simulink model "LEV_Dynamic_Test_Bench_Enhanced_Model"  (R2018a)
settings: Solver=VariableStepAuto  StartTime=0  StopTime=100  RelTol=1e-3
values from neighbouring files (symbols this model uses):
  Anglog_Input_Max = 10    [Panda_BEVintage_VPE_S_Data_Enhanced_Model.m]    (also in ParameterInitializationFileFinal.m = 3; Panda_BEVintage_VPE_S_Data_CodeGen_Model.m)
  Anglog_Input_Min = -10    [Panda_BEVintage_VPE_S_Data_Enhanced_Model.m]    (also in ParameterInitializationFileFinal.m = 0; Panda_BEVintage_VPE_S_Data_CodeGen_Model.m)
  Anglog_Output_Max = 10    [Panda_BEVintage_VPE_S_Data_Enhanced_Model.m]    (also in Panda_BEVintage_VPE_S_Data_CodeGen_Model.m)
  Anglog_Output_Min = -10    [Panda_BEVintage_VPE_S_Data_Enhanced_Model.m]    (also in Panda_BEVintage_VPE_S_Data_CodeGen_Model.m)
  Bits = 16    [Panda_BEVintage_VPE_S_Data_Enhanced_Model.m]    (also in ParameterInitializationFileFinal.m = 12; Panda_BEVintage_VPE_S_Data_CodeGen_Model.m)
  c_1 = 0    [Panda_BEVintage_VPE_S_Data_Enhanced_Model.m]    (also in Panda_BEVintage_VPE_S_Data_CodeGen_Model.m)
  FOH_Time = 0.001    [Panda_BEVintage_VPE_S_Data_Enhanced_Model.m]    (also in Panda_BEVintage_VPE_S_Data_CodeGen_Model.m)
  Full_BTrq_Range = Max_BTrq-Min_BTrq    (= 132)    [Panda_BEVintage_VPE_S_Data_Enhanced_Model.m]    (also in Panda_BEVintage_VPE_S_Data_CodeGen_Model.m)
  Full_Scale_Reading = Anglog_Input_Max-Anglog_Input_Min    (= 20)    [Panda_BEVintage_VPE_S_Data_Enhanced_Model.m]    (also in ParameterInitializationFileFinal.m = 3; Panda_BEVintage_VPE_S_Data_CodeGen_Model.m)
  Full_Speed_Range = Max_Speed-Min_Speed    (= 2513.27412287)    [Panda_BEVintage_VPE_S_Data_Enhanced_Model.m]    (also in Panda_BEVintage_VPE_S_Data_CodeGen_Model.m)
  g = 9.81    [Panda_BEVintage_VPE_S_Data_Enhanced_Model.m]    (also in Panda_BEVintage_VPE_S_Data_CodeGen_Model.m)
  m_e = 1.0359e+03    (= 1035.9)    [Panda_BEVintage_VPE_S_Data_Enhanced_Model.m]    (also in Panda_BEVintage_VPE_S_Data_CodeGen_Model.m)
  Max_BTrq = T_m_max    (= 66)    [Panda_BEVintage_VPE_S_Data_Enhanced_Model.m]    (also in Panda_BEVintage_VPE_S_Data_CodeGen_Model.m)
  Max_Speed = 400*pi    (= 1256.63706144)    [Panda_BEVintage_VPE_S_Data_Enhanced_Model.m]    (also in Panda_BEVintage_VPE_S_Data_CodeGen_Model.m)
  MaxInputBTrq = 5    [Panda_BEVintage_VPE_S_Data_Enhanced_Model.m]    (also in Panda_BEVintage_VPE_S_Data_CodeGen_Model.m)
  MaxOutputSpeedSensor = 5    [Panda_BEVintage_VPE_S_Data_Enhanced_Model.m]    (also in Panda_BEVintage_VPE_S_Data_CodeGen_Model.m)
  Min_BTrq = -T_m_max    (= -66)    [Panda_BEVintage_VPE_S_Data_Enhanced_Model.m]    (also in Panda_BEVintage_VPE_S_Data_CodeGen_Model.m)
  Min_Speed = -400*pi    (= -1256.63706144)    [Panda_BEVintage_VPE_S_Data_Enhanced_Model.m]    (also in Panda_BEVintage_VPE_S_Data_CodeGen_Model.m)
  MinInputBTrq = -5    [Panda_BEVintage_VPE_S_Data_Enhanced_Model.m]    (also in Panda_BEVintage_VPE_S_Data_CodeGen_Model.m)
  MinOutputSpeedSensor = -5    [Panda_BEVintage_VPE_S_Data_Enhanced_Model.m]    (also in Panda_BEVintage_VPE_S_Data_CodeGen_Model.m)
  r_e = 0.27    [Panda_BEVintage_VPE_S_Data_Enhanced_Model.m]    (also in Panda_BEVintage_VPE_S_Data_CodeGen_Model.m)
  Sampling_Time = 0.0001    [Panda_BEVintage_VPE_S_Data_Enhanced_Model.m]    (also in ParameterInitializationFileFinal.m = 0.01; Panda_BEVintage_VPE_S_Data_CodeGen_Model.m)
  T_m_max = 66    [Panda_BEVintage_VPE_S_Data_Enhanced_Model.m]    (also in Panda_BEVintage_VPE_S_Data_CodeGen_Model.m)
  T_r = 8.67    [Panda_BEVintage_VPE_S_Data_Enhanced_Model.m]    (also in Panda_BEVintage_VPE_S_Data_CodeGen_Model.m)
  ZOH_Time = 0.0001    [Panda_BEVintage_VPE_S_Data_Enhanced_Model.m]    (also in Panda_BEVintage_VPE_S_Data_CodeGen_Model.m)
undefined symbols (not defined in the file or in its folder): m, s, seconds
libraries: simulink x3, autolibmappedmotor x2, autolibshared x2, autolibsharedcoupling x1

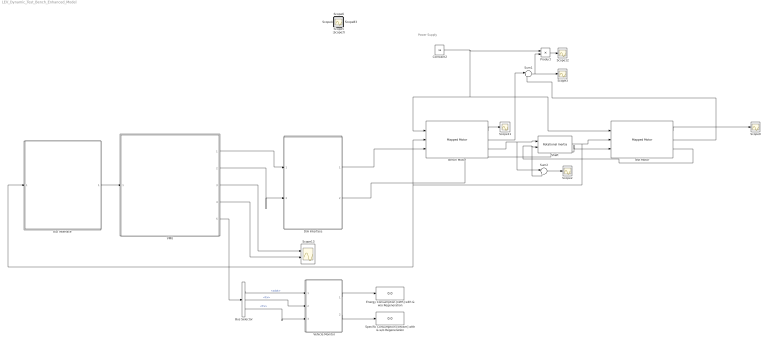
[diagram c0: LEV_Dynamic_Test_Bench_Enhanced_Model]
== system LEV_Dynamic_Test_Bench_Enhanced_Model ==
  note: Power Supply
  "A/D Interface " : Subsystem
  Bench Motor : autolibmappedmotor/Mapped Motor  port_config=Speed  param_by=Maximum torque and power  w_t=[ 0 375 750 800 ]  T_t=[0.09 0.08 0.07 0]  torque_max=T_m_max  power_max=P_m_max  Tc=tau_m  param_loss=Single efficiency measurement  eff=eta_n  w_eff=w_n  T_eff=T_m_n  Piron=Pl_iron  Pbase=Pl_eln  w_eff_bp=[-8000 -4000 0 4000 8000]  T_eff_bp=[0 0.03 0.06 0.09]  losses_table=[1 2;3 4]  efficiency_table=[95 95 95 95; 95 95 95 95; 95 95 95 95; 95 95 95 95; 95 95 95 95]  J=5e-6  b=1e-5  omega_o=0  T_t_extended=[0 0.07 0.08 0.09 0.08 0.07 0]  w_t_extended=[-800 -750 -375 0 375 750 800]  KLossIron=0  KLossCopper=0.68708  x_w_eff_vec=[-400 0 400]  x_T_eff_vec=[-20 0 20]  x_losses_mat=[4 3 4;2 1 2;4 3 4]  aMode=aMode
  Bus Selector : BusSelector  OutputSignals=BdyFrm.Cg.Vel.xdot,BdyFrm.Forces.Ext.Fx,BdyFrm.Forces.Drag.Fx
  Constant2 : Constant  Value=96
  D/A Interface : Subsystem
  Energy Consumption [kWh] with & w/o Regeneration : Display
  Product : Product
  Scope{,1..12,18} (14 alike) : Scope
  Scope13 : Scope  NumInputPorts=2
  Shaft : autolibsharedcoupling/Rotational Inertia  port_config=Simulink  J=.01  b=.001  omega_o=0  externJ=off  blkID=0  aMode=1
  Specific Consumption [kW/km] with & w/o Regeneration : Display
  Sum1 : Sum  Inputs=|++
  Sum2 : Sum  Inputs=|++
  Test Motor : autolibmappedmotor/Mapped Motor  port_config=Speed  param_by=Maximum torque and power  w_t=[ 0 375 750 800 ]  T_t=[0.09 0.08 0.07 0]  torque_max=T_m_max  power_max=P_m_max  Tc=tau_m  param_loss=Single efficiency measurement  eff=eta_n  w_eff=w_n  T_eff=T_m_n  Piron=Pl_iron  Pbase=Pl_eln  w_eff_bp=[-8000 -4000 0 4000 8000]  T_eff_bp=[0 0.03 0.06 0.09]  losses_table=[1 2;3 4]  efficiency_table=[95 95 95 95; 95 95 95 95; 95 95 95 95; 95 95 95 95; 95 95 95 95]  J=5e-6  b=1e-5  omega_o=0  T_t_extended=[0 0.07 0.08 0.09 0.08 0.07 0]  w_t_extended=[-800 -750 -375 0 375 750 800]  KLossIron=0  KLossCopper=0.68708  x_w_eff_vec=[-400 0 400]  x_T_eff_vec=[-20 0 20]  x_losses_mat=[4 3 4;2 1 2;4 3 4]  aMode=aMode
  VMU : Subsystem
  Vehicle Monitor : Subsystem
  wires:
  Test Motor/3 -> Shaft/2, Sum2/2
  Bench Motor/3 -> Sum2/1, Shaft/1
  Constant2/1 -> Bench Motor/1, Test Motor/1, Product/1
  Shaft/1 -> "A/D Interface "/1(ShaftSpeed), Bench Motor/2, Test Motor/2
  Test Motor/2 -> Sum1/2
  Sum1/1 -> Product/2, Scope3/1
  Bench Motor/2 -> Sum1/1
  Sum2/1 -> Scope2/1
  Bench Motor/1 -> Scope11/1
  Test Motor/1 -> Scope9/1
  Product/1 -> Scope12/1
  Bus Selector/1 -> Vehicle Monitor/1(In1)  "<xdot>"
  Bus Selector/3 -> Vehicle Monitor/3(In3)  "<Fx>"
  Bus Selector/2 -> Vehicle Monitor/2(In2)  "<Fx>"
  Vehicle Monitor/1(Out1) -> Energy Consumption [kWh] with & w/o Regeneration/1
  Vehicle Monitor/2(Out2) -> Specific Consumption [kW/km] with & w/o Regeneration/1
  D/A Interface/1("BenchTrqCMD ") -> Bench Motor/3
  D/A Interface/2("MotorTrqCMD ") -> Test Motor/3
  VMU/1(BenchTrqCMD) -> D/A Interface/1(DigitalBenchTrqCMD)
  VMU/2(MotorTrqCMD) -> D/A Interface/2(DigitalMotorTrqCMD)
  VMU/3(Speed [m/s]) -> Scope13/1
  VMU/4(ForceTot) -> Scope13/2
  VMU/5(Out5) -> Bus Selector/1
  "A/D Interface "/1("AverageShaftSpeedDigitalSignal ") -> VMU/1("AverageShaftSpeedDigitalSignal ")

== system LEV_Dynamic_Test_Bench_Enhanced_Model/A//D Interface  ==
  ShaftSpeed : Inport
  ADC BOUNDARY : Subsystem
  DigitalSignalPreProcessing : Subsystem
  LinearTransducer : Subsystem
  Signal Averaging Block : Subsystem
  Signal Scaling to Adapt Target Input Dynamics : Subsystem
  "AverageShaftSpeedDigitalSignal " : Outport
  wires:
  Signal Scaling to Adapt Target Input Dynamics/1(SignalScaledToTargetDynamics -10 to +10 [V]) -> ADC BOUNDARY/1(ShaftSpeedSignal)
  ADC BOUNDARY/1(ShaftSpeedDigitalSignal) -> DigitalSignalPreProcessing/1(ShaftSpeedDigitalSignal)
  ShaftSpeed/1 -> LinearTransducer/1("ShaftSpeed ")
  LinearTransducer/1(SpeedSensorOutputVoltage -5 to +5 [V]) -> Signal Scaling to Adapt Target Input Dynamics/1("SpeedSensorOutputVoltage ")
  DigitalSignalPreProcessing/1("ShaftSpeedDigitalSignal ") -> Signal Averaging Block/1("ShaftSpeedDigitalSignal ")
  Signal Averaging Block/1("AverageShaftSpeedDigitalSignal ") -> "AverageShaftSpeedDigitalSignal "/1

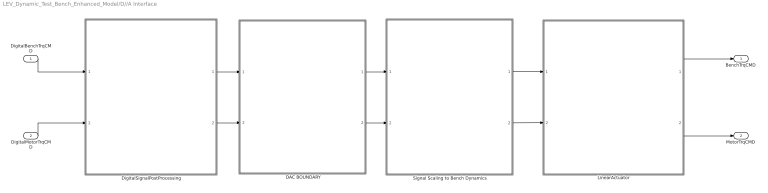
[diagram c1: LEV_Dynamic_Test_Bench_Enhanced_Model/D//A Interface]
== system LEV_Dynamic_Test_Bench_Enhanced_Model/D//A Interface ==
  DigitalBenchTrqCMD : Inport
  DigitalMotorTrqCMD : Inport  Port=2
  DAC BOUNDARY : Subsystem
  DigitalSignalPostProcessing : Subsystem
  LinearActuator : Subsystem
  Signal Scaling to Bench Dynamics : Subsystem
  "BenchTrqCMD " : Outport
  "MotorTrqCMD " : Outport  Port=2
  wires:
  DAC BOUNDARY/1(AnalogBenchTrqCMD -10 to +10 V) -> Signal Scaling to Bench Dynamics/1(" AnalogBenchTrqCMD -10 to +10 V ")
  DAC BOUNDARY/2("AnalogMotorTrqCMD -10 to +10 V ") -> Signal Scaling to Bench Dynamics/2("AnalogMotorTrqCMD -10 to +10 V ")
  DigitalMotorTrqCMD/1 -> DigitalSignalPostProcessing/2(MotorTrqCMD)
  DigitalBenchTrqCMD/1 -> DigitalSignalPostProcessing/1(BenchTrqCMD)
  LinearActuator/1(BenchTrqCMD) -> "BenchTrqCMD "/1
  Signal Scaling to Bench Dynamics/1(BenchTrqCmdInVolts) -> LinearActuator/1(BenchTrqCmdInVolts)
  DigitalSignalPostProcessing/1(BenchTrqCMD16Bits) -> DAC BOUNDARY/1(BenchTrqCMD16Bits)
  DigitalSignalPostProcessing/2(MotorTrqCMD16Bits) -> DAC BOUNDARY/2(MotorTrqCMD16Bits)
  Signal Scaling to Bench Dynamics/2(MotorTrqCmdInVolts) -> LinearActuator/2(MotorTrqCmdInVolts)
  LinearActuator/2(MotorTrqCMD) -> "MotorTrqCMD "/1

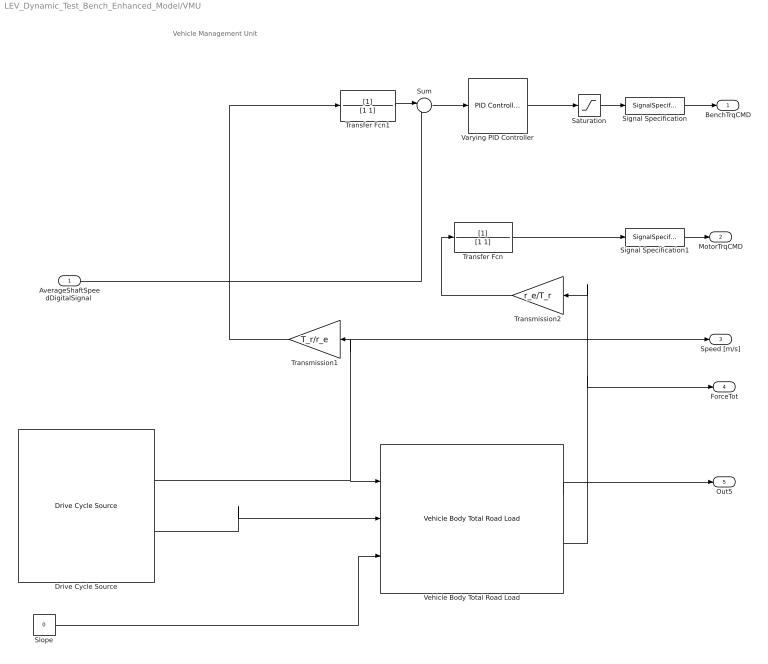
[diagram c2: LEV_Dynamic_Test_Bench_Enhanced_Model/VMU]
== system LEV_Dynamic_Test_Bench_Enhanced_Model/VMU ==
  note: Vehicle Management Unit
  "AverageShaftSpeedDigitalSignal " : Inport
  Drive Cycle Source : autolibshared/Drive Cycle Source  cycleVar=FTP75  fileVar=cycleFTP75.mat  tfinal="2474  seconds"  cycleRepeat=off  outAccPort=on  outGearPort=off  gearList=No gear data  t_wot1=5  xdot_woto=0  xdot_wot1=10  t_wot2=20  xdot_wot2=0  t_wotend=30  srcUnit=m/s  outUnit=m/s  srcAccUnit=m/s/s  outAccUnit=m/s^2  dt=0  aMode=aMode
  Saturation : Saturate  UpperLimit=T_m_max  LowerLimit=-T_m_max
  Signal Specification : SignalSpecification  Unit=N*m
  Signal Specification1 : SignalSpecification  Unit=N*m
  Slope : Constant  Value=0
  Sum : Sum  Inputs=|+-
  Transfer Fcn : TransferFcn  Denominator=[1 1]
  Transfer Fcn1 : TransferFcn  Denominator=[1 1]
  Transmission1 : Gain  Gain=T_r/r_e
  Transmission2 : Gain  Gain=r_e/T_r
  Varying PID Controller : simulink/Continuous/PID Controller  Controller=PI  TimeDomain=Continuous-time  SampleTime=-1  IntegratorMethod=Forward Euler  FilterMethod=Forward Euler  Form=Parallel  UseFilter=on  ControllerParametersSource=internal  P=.5  I=.5  D=0  N=100  InitialConditionSource=internal  InitialConditionForIntegrator=0  InitialConditionForFilter=0  ExternalReset=none  LimitOutput=off  UpperSaturationLimit=inf  LowerSaturationLimit=-inf  LinearizeAsGain=on  AntiWindupMode=none  Kb=1  TrackingMode=off  Kt=1  PParamMin=[]  PParamMax=[]  IParamMin=[]  IParamMax=[]  DParamMin=[]  DParamMax=[]  NParamMin=[]  NParamMax=[]  KbParamMin=[]  KbParamMax=[]  KtParamMin=[]  KtParamMax=[]  POutMin=[]  POutMax=[]  IOutMin=[]  IOutMax=[]  DOutMin=[]  DOutMax=[]  NOutMin=[]  NOutMax=[]  KbOutMin=[]  KbOutMax=[]  KtOutMin=[]  KtOutMax=[]  IntegratorOutMin=[]  IntegratorOutMax=[]  FilterOutMin=[]  FilterOutMax=[]  SumOutMin=[]  SumOutMax=[]  SumI1OutMin=[]  SumI1OutMax=[]  SumI2OutMin=[]  SumI2OutMax=[]  SumI3OutMin=[]  SumI3OutMax=[]  SumDOutMin=[]  SumDOutMax=[]  SaturationOutMin=[]  SaturationOutMax=[]  IntegratorContinuousStateAttributes=''  IntegratorStateMustResolveToSignalObject=off  IntegratorRTWStateStorageClass=Auto  FilterContinuousStateAttributes=''  FilterStateMustResolveToSignalObject=off  FilterRTWStateStorageClass=Auto  DifferentiatorICPrevScaledInput=0  DifferentiatorOutMin=[]  DifferentiatorOutMax=[]  InitialConditionSetting=State (most efficient)  FilterDiffOutCoefMin=[]  FilterDiffOutCoefMax=[]  SumDenOutMin=[]  SumDenOutMax=[]  SumNumOutMin=[]  SumNumOutMax=[]  ReciprocalOutMin=[]  ReciprocalOutMax=[]  DivideOutMin=[]  DivideOutMax=[]  TunerSelectOption=Transfer Function Based (PID Tuner App)
  Vehicle Body Total Road Load : autolibshared/Vehicle Body Total Road Load  VariantControl=SL1dof  input_type=Kinematic  aMode=aMode  m=m_e  a=c_0  b=c_1  c=c_2  g=g  xdot_o=0
  BenchTrqCMD : Outport
  MotorTrqCMD : Outport  Port=2
  Speed [m/s] : Outport  Port=3
  ForceTot : Outport  Port=4
  Out5 : Outport  Port=5
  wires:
  Vehicle Body Total Road Load/2 -> Transmission2/1, ForceTot/1
  Transmission2/1 -> Transfer Fcn/1
  Transmission1/1 -> Transfer Fcn1/1
  Transfer Fcn1/1 -> Sum/1
  Slope/1 -> Vehicle Body Total Road Load/3
  "AverageShaftSpeedDigitalSignal "/1 -> Sum/2
  Sum/1 -> Varying PID Controller/1
  Varying PID Controller/1 -> Saturation/1
  Transfer Fcn/1 -> Signal Specification1/1
  Vehicle Body Total Road Load/1 -> Out5/1
  Saturation/1 -> Signal Specification/1
  Signal Specification/1 -> BenchTrqCMD/1
  Signal Specification1/1 -> MotorTrqCMD/1
  Drive Cycle Source/1 -> Vehicle Body Total Road Load/1, Transmission1/1, Speed [m/s]/1
  Drive Cycle Source/2 -> Vehicle Body Total Road Load/2

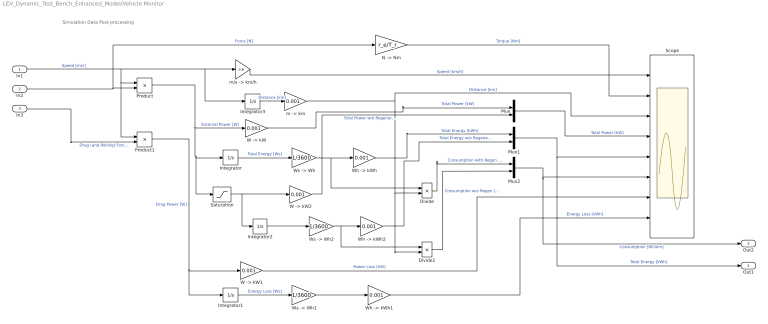
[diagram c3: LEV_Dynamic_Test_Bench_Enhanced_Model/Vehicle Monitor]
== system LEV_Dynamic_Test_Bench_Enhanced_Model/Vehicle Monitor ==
  note: Simulation Data Post-processing
  In1 : Inport
  In2 : Inport  Port=2
  In3 : Inport  Port=3
  Divide : Product  Inputs=*/
  Divide1 : Product  Inputs=*/
  Integrator{,1..3} (4 alike) : Integrator
  Mux : Mux  Inputs=2
  Mux1 : Mux  Inputs=2
  Mux2 : Mux  Inputs=2
  "N -> Nm" : Gain  Gain=r_e/T_r
  Product : Product
  Product1 : Product
  Saturation : Saturate  UpperLimit=inf  LowerLimit=0
  Scope : Scope  NumInputPorts=8
  "W -> kW" : Gain  Gain=0.001
  "W -> kW1" : Gain  Gain=0.001
  "W -> kW2" : Gain  Gain=0.001
  "Wh -> kWh" : Gain  Gain=0.001
  "Wh -> kWh1" : Gain  Gain=0.001
  "Wh -> kWh2" : Gain  Gain=0.001
  "Ws -> Wh" : Gain  Gain=1/3600
  "Ws -> Wh1" : Gain  Gain=1/3600
  "Ws -> Wh2" : Gain  Gain=1/3600
  "m -> km" : Gain  Gain=0.001
  "m/s -> km/h" : Gain  Gain=3.6
  Out1 : Outport
  Out2 : Outport  Port=2
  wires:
  Divide/1 -> Mux2/1  "Consumption with Regen [Wh/km]"
  "Wh -> kWh1"/1 -> Scope/8  "Energy Loss [kWh]"
  Saturation/1 -> Integrator2/1, "W -> kW2"/1
  "Wh -> kWh2"/1 -> Mux1/2  "Total Energy w/o Regeneration [kWh]"
  Mux1/1 -> Out1/1, Scope/5  "Total Energy [kWh]"
  "W -> kW"/1 -> Mux/1  "Total Power [kW]"
  Divide1/1 -> Mux2/2  "Consumption w/o Regen [Wh/km]"
  "Wh -> kWh"/1 -> Mux1/1  "Total Energy [kWh]"
  "W -> kW1"/1 -> Scope/7  "Power Loss [kW]"
  Integrator/1 -> "Ws -> Wh"/1  "Total Energy [Ws]"
  Integrator1/1 -> "Ws -> Wh1"/1  "Energy Loss [Ws]"
  "Ws -> Wh2"/1 -> Divide1/1, "Wh -> kWh2"/1
  Product1/1 -> Integrator1/1, "W -> kW1"/1  "Drag Power [W]"
  "N -> Nm"/1 -> Scope/2  "Torque [Nm]"
  Mux/1 -> Scope/4  "Total Power [kW]"
  "W -> kW2"/1 -> Mux/2  "Total Power w/o Regeneration [kW]"
  Mux2/1 -> Out2/1, Scope/6  "Consumption [Wh/km]"
  Integrator2/1 -> "Ws -> Wh2"/1
  "Ws -> Wh1"/1 -> "Wh -> kWh1"/1
  "m -> km"/1 -> Scope/3, Divide1/2, Divide/2  "Distance [km]"
  In2/1 -> "N -> Nm"/1, Product/2  "Force [N]"
  Product/1 -> Saturation/1, Integrator/1, "W -> kW"/1  "External Power [W]"
  "Ws -> Wh"/1 -> Divide/1, "Wh -> kWh"/1
  Integrator3/1 -> "m -> km"/1  "Distance [km]"
  "m/s -> km/h"/1 -> Scope/1  "Speed [km/h]"
  In1/1 -> Product1/1, Product/1, "m/s -> km/h"/1, Integrator3/1  "Speed [m/s]"
  In3/1 -> Product1/2  "Drag (and Rolling) Force [N]"

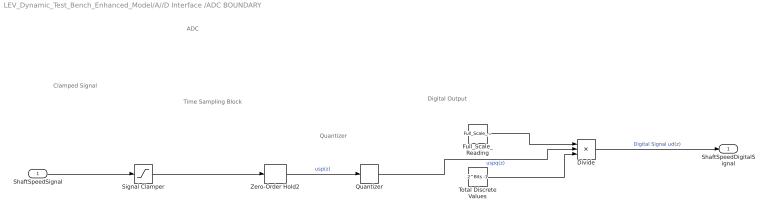
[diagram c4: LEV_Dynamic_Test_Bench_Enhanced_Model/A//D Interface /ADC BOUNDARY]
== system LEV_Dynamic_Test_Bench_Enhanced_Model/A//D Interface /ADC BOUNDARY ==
  note: Quantizer
  note: Time Sampling Block
  note: Digital Output
  note: Clamped Signal
  note: ADC
  ShaftSpeedSignal : Inport
  Divide : Product  Inputs=/**
  Full_Scale_Reading : Constant  Value=Full_Scale_Reading
  Quantizer : Quantizer  QuantizationInterval=Full_Scale_Reading/(2^Bits-1 )
  Signal Clamper : Saturate  UpperLimit=Anglog_Input_Max  LowerLimit=Anglog_Input_Min
  Total Discrete Values : Constant  Value=2^Bits -1
  Zero-Order Hold2 : ZeroOrderHold  SampleTime=Sampling_Time
  ShaftSpeedDigitalSignal : Outport
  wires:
  Signal Clamper/1 -> Zero-Order Hold2/1
  ShaftSpeedSignal/1 -> Signal Clamper/1
  Full_Scale_Reading/1 -> Divide/1
  Total Discrete Values/1 -> Divide/3
  Quantizer/1 -> Divide/2  "uspq(z)"
  Divide/1 -> ShaftSpeedDigitalSignal/1  "Digital Signal ud(z)"
  Zero-Order Hold2/1 -> Quantizer/1  "usp(z)"

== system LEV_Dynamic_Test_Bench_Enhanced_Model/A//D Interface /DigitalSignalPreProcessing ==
  ShaftSpeedDigitalSignal : Inport
  ScalingToSignalValues : Subsystem
  "ShaftSpeedDigitalSignal " : Outport
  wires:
  ShaftSpeedDigitalSignal/1 -> ScalingToSignalValues/1(ShaftSpeedDigitalSignal)
  ScalingToSignalValues/1("ShaftSpeedDigitalSignal ") -> "ShaftSpeedDigitalSignal "/1

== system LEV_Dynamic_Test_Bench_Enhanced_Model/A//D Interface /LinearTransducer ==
  "ShaftSpeed " : Inport
  Add : Sum
  Offset Term c : Subsystem
  Product : Product
  Scaling Coefficient m : Subsystem
  Signal Specification : SignalSpecification  Unit=V
  SpeedSensorOutputVoltage -5 to +5 [V] : Outport
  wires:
  Add/1 -> Signal Specification/1
  Scaling Coefficient m/1(Scaling Coefficient m) -> Product/1, Offset Term c/1(Scaling Coefficent m)
  Product/1 -> Add/2
  Offset Term c/1("Offset Term c ") -> Add/1
  "ShaftSpeed "/1 -> Product/2
  Signal Specification/1 -> SpeedSensorOutputVoltage -5 to +5 [V]/1

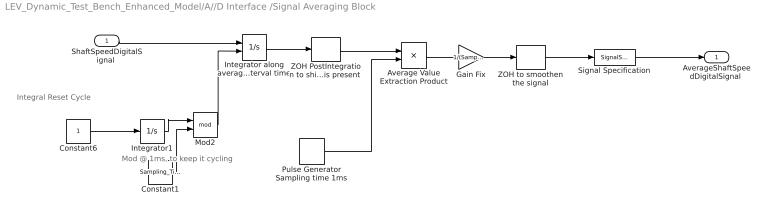
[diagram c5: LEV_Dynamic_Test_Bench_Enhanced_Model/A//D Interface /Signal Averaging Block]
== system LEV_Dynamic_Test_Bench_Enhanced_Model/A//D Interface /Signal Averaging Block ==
  note: Mod @ 1ms, to keep it cycling
  note: Integral Reset Cycle
  "ShaftSpeedDigitalSignal " : Inport
  Average Value Extraction Product : Product
  Constant1 : Constant  Value=Sampling_Time*10
  Constant6 : Constant
  Gain Fix : Gain  Gain=1/(Sampling_Time*10)
  Integrator along averaging interval time : Integrator  ExternalReset=rising
  Integrator1 : Integrator
  Mod2 : Math  Operator=mod
  Pulse Generator Sampling time 1ms : DiscretePulseGenerator  PulseType=Time based  Period=Sampling_Time*10
  Signal Specification : SignalSpecification  Unit=rad/s
  "ZOH PostIntegration to shift left or delay by one sample time, so that at the sample time of extraction of avg value,signal is present " : ZeroOrderHold  SampleTime=-1
  ZOH to smoothen the signal : ZeroOrderHold  SampleTime=Sampling_Time*10
  "AverageShaftSpeedDigitalSignal " : Outport
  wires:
  Gain Fix/1 -> ZOH to smoothen the signal/1
  Integrator along averaging interval time/1 -> "ZOH PostIntegration to shift left or delay by one sample time, so that at the sample time of extraction of avg value,signal is present "/1
  Constant1/1 -> Mod2/2
  Average Value Extraction Product/1 -> Gain Fix/1
  Integrator1/1 -> Mod2/1
  "ShaftSpeedDigitalSignal "/1 -> Integrator along averaging interval time/1
  "ZOH PostIntegration to shift left or delay by one sample time, so that at the sample time of extraction of avg value,signal is present "/1 -> Average Value Extraction Product/1
  Mod2/1 -> Integrator along averaging interval time/2
  ZOH to smoothen the signal/1 -> Signal Specification/1
  Pulse Generator Sampling time 1ms/1 -> Average Value Extraction Product/2
  Signal Specification/1 -> "AverageShaftSpeedDigitalSignal "/1
  Constant6/1 -> Integrator1/1

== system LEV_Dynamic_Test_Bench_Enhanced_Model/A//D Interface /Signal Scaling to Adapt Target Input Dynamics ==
  "SpeedSensorOutputVoltage " : Inport
  Add : Sum
  Offset Term c : Subsystem
  Product : Product
  Scaling Coefficient m : Subsystem
  Signal Specification : SignalSpecification  Unit=V
  SignalScaledToTargetDynamics -10 to +10 [V] : Outport
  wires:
  Scaling Coefficient m/1(Scaling Coefficient m) -> Product/1, Offset Term c/1(Scaling Coefficent m)
  "SpeedSensorOutputVoltage "/1 -> Product/2
  Product/1 -> Add/2
  Offset Term c/1("Offset Term c ") -> Add/1
  Add/1 -> Signal Specification/1
  Signal Specification/1 -> SignalScaledToTargetDynamics -10 to +10 [V]/1

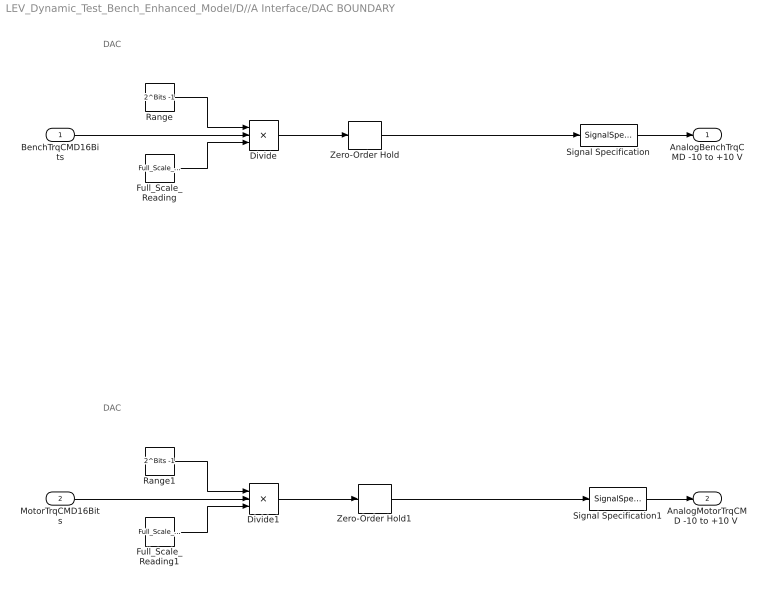
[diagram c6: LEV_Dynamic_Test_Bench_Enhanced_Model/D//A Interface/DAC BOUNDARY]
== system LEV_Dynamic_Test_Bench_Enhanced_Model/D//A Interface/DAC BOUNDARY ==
  note: DAC
  note: DAC
  BenchTrqCMD16Bits : Inport
  MotorTrqCMD16Bits : Inport  Port=2
  Divide : Product  Inputs=/**
  Divide1 : Product  Inputs=/**
  Full_Scale_Reading : Constant  Value=Full_Scale_Reading
  Full_Scale_Reading1 : Constant  Value=Full_Scale_Reading
  Range : Constant  Value=2^Bits -1
  Range1 : Constant  Value=2^Bits -1
  Signal Specification : SignalSpecification  Unit=V
  Signal Specification1 : SignalSpecification  Unit=V
  Zero-Order Hold : ZeroOrderHold  SampleTime=ZOH_Time
  Zero-Order Hold1 : ZeroOrderHold  SampleTime=ZOH_Time
  AnalogBenchTrqCMD -10 to +10 V : Outport
  "AnalogMotorTrqCMD -10 to +10 V " : Outport  Port=2
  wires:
  Range/1 -> Divide/1
  Full_Scale_Reading/1 -> Divide/3
  BenchTrqCMD16Bits/1 -> Divide/2
  Divide/1 -> Zero-Order Hold/1
  Full_Scale_Reading1/1 -> Divide1/3
  Divide1/1 -> Zero-Order Hold1/1
  MotorTrqCMD16Bits/1 -> Divide1/2
  Range1/1 -> Divide1/1
  Signal Specification1/1 -> "AnalogMotorTrqCMD -10 to +10 V "/1
  Signal Specification/1 -> AnalogBenchTrqCMD -10 to +10 V/1
  Zero-Order Hold1/1 -> Signal Specification1/1
  Zero-Order Hold/1 -> Signal Specification/1

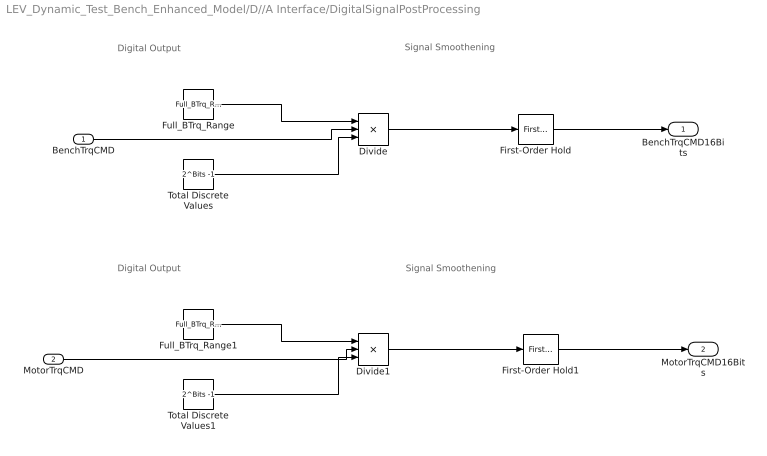
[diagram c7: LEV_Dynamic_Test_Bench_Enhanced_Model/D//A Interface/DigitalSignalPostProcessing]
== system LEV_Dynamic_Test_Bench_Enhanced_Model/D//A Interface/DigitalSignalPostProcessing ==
  note: Digital Output
  note: Digital Output
  note: Signal Smoothening
  note: Signal Smoothening
  BenchTrqCMD : Inport
  MotorTrqCMD : Inport  Port=2
  Divide : Product  Inputs=/**
  Divide1 : Product  Inputs=/**
  First-Order Hold : simulink/Discrete/First-Order Hold  DisableCoverage=on  Ts=FOH_Time
  First-Order Hold1 : simulink/Discrete/First-Order Hold  DisableCoverage=on  Ts=FOH_Time
  Full_BTrq_Range : Constant  Value=Full_BTrq_Range
  Full_BTrq_Range1 : Constant  Value=Full_BTrq_Range
  Total Discrete Values : Constant  Value=2^Bits -1
  Total Discrete Values1 : Constant  Value=2^Bits -1
  BenchTrqCMD16Bits : Outport
  MotorTrqCMD16Bits : Outport  Port=2
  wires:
  Divide/1 -> First-Order Hold/1
  BenchTrqCMD/1 -> Divide/2
  Full_BTrq_Range/1 -> Divide/1
  Total Discrete Values/1 -> Divide/3
  Total Discrete Values1/1 -> Divide1/3
  MotorTrqCMD/1 -> Divide1/2
  Divide1/1 -> First-Order Hold1/1
  Full_BTrq_Range1/1 -> Divide1/1
  First-Order Hold/1 -> BenchTrqCMD16Bits/1
  First-Order Hold1/1 -> MotorTrqCMD16Bits/1

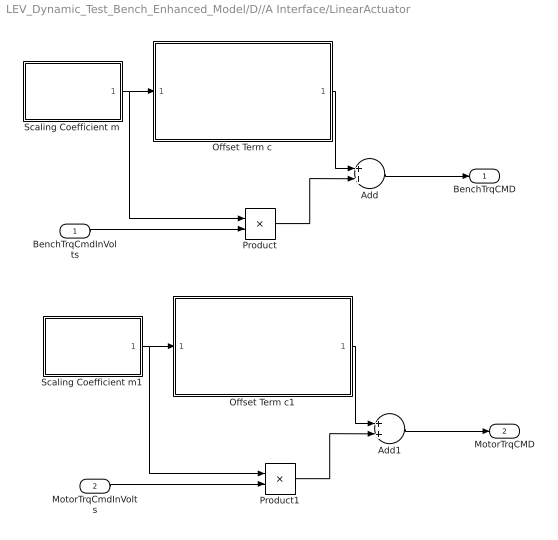
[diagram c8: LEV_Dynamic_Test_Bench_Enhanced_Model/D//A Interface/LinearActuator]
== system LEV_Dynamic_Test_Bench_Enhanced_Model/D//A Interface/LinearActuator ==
  BenchTrqCmdInVolts : Inport
  MotorTrqCmdInVolts : Inport  Port=2
  Add : Sum
  Add1 : Sum
  Offset Term c : Subsystem
  Offset Term c1 : Subsystem
  Product : Product
  Product1 : Product
  Scaling Coefficient m : Subsystem
  Scaling Coefficient m1 : Subsystem
  BenchTrqCMD : Outport
  MotorTrqCMD : Outport  Port=2
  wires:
  Add/1 -> BenchTrqCMD/1
  Scaling Coefficient m/1(Scaling Coefficient m) -> Product/1, Offset Term c/1(Scaling Coefficent m)
  Product/1 -> Add/2
  Offset Term c/1("Offset Term c ") -> Add/1
  BenchTrqCmdInVolts/1 -> Product/2
  MotorTrqCmdInVolts/1 -> Product1/2
  Scaling Coefficient m1/1(Scaling Coefficient m) -> Product1/1, Offset Term c1/1(Scaling Coefficent m)
  Product1/1 -> Add1/2
  Add1/1 -> MotorTrqCMD/1
  Offset Term c1/1("Offset Term c ") -> Add1/1

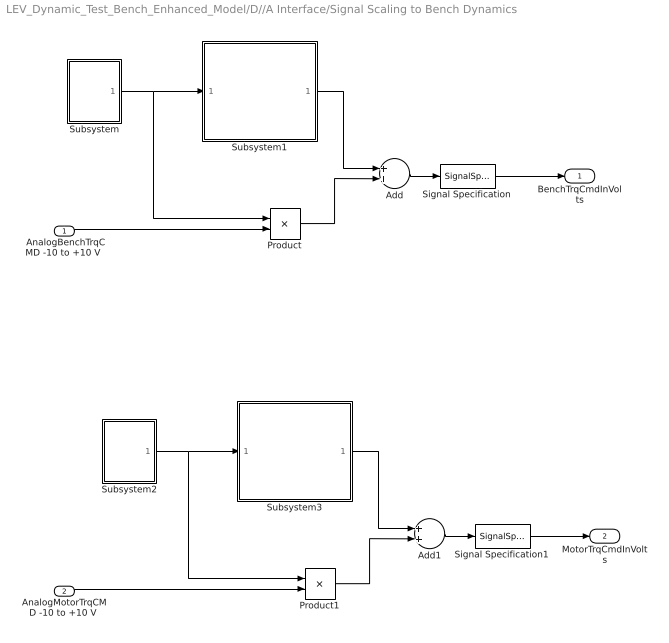
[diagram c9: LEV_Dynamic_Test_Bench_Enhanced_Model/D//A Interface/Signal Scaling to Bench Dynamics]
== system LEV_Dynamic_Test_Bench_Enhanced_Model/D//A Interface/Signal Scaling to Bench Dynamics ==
  " AnalogBenchTrqCMD -10 to +10 V " : Inport
  "AnalogMotorTrqCMD -10 to +10 V " : Inport  Port=2
  Add : Sum
  Add1 : Sum
  Product : Product
  Product1 : Product
  Signal Specification : SignalSpecification  Unit=V
  Signal Specification1 : SignalSpecification  Unit=V
  Subsystem : Subsystem
  Subsystem1 : Subsystem
  Subsystem2 : Subsystem
  Subsystem3 : Subsystem
  BenchTrqCmdInVolts : Outport
  MotorTrqCmdInVolts : Outport  Port=2
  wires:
  Product/1 -> Add/2
  Add/1 -> Signal Specification/1
  Subsystem/1("Gradient ") -> Product/1, Subsystem1/1("Gradient ")
  Subsystem1/1("Offset ") -> Add/1
  " AnalogBenchTrqCMD -10 to +10 V "/1 -> Product/2
  Add1/1 -> Signal Specification1/1
  "AnalogMotorTrqCMD -10 to +10 V "/1 -> Product1/2
  Subsystem3/1("Offset ") -> Add1/1
  Subsystem2/1("Gradient ") -> Product1/1, Subsystem3/1("Gradient ")
  Product1/1 -> Add1/2
  Signal Specification1/1 -> MotorTrqCmdInVolts/1
  Signal Specification/1 -> BenchTrqCmdInVolts/1

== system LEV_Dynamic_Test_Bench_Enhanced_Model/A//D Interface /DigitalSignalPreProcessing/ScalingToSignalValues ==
  ShaftSpeedDigitalSignal : Inport
  Divide : Product  Inputs=/**
  Full_Scale_Reading : Constant  Value=Full_Speed_Range
  Signal Specification : SignalSpecification  Unit=rad/s
  Values : Constant  Value=2^Bits -1
  "ShaftSpeedDigitalSignal " : Outport
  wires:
  ShaftSpeedDigitalSignal/1 -> Divide/2
  Values/1 -> Divide/1
  Divide/1 -> Signal Specification/1  "ShaftSpeedDigitalSignal"
  Full_Scale_Reading/1 -> Divide/3
  Signal Specification/1 -> "ShaftSpeedDigitalSignal "/1

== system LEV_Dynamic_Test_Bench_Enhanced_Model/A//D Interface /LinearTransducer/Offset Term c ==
  Scaling Coefficent m : Inport
  MinOutputSpeedSensor : Constant  Value=MinOutputSpeedSensor
  Min_Speed : Constant  Value=Min_Speed
  Product : Product
  Subtract2 : Sum  Inputs=+-
  "Offset Term c " : Outport
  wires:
  Min_Speed/1 -> Product/1
  Scaling Coefficent m/1 -> Product/2
  Product/1 -> Subtract2/2
  Subtract2/1 -> "Offset Term c "/1
  MinOutputSpeedSensor/1 -> Subtract2/1

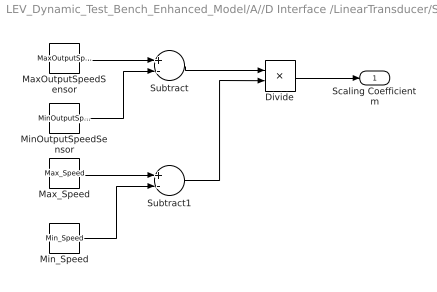
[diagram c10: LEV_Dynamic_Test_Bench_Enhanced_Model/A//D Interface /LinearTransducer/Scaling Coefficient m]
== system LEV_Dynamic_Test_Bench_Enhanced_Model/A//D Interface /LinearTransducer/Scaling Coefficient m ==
  Divide : Product  Inputs=*/
  MaxOutputSpeedSensor : Constant  Value=MaxOutputSpeedSensor
  Max_Speed : Constant  Value=Max_Speed
  MinOutputSpeedSensor : Constant  Value=MinOutputSpeedSensor
  Min_Speed : Constant  Value=Min_Speed
  Subtract : Sum  Inputs=+-
  Subtract1 : Sum  Inputs=+-
  Scaling Coefficient m : Outport
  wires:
  Divide/1 -> Scaling Coefficient m/1
  Subtract1/1 -> Divide/2
  Subtract/1 -> Divide/1
  MinOutputSpeedSensor/1 -> Subtract/2
  Min_Speed/1 -> Subtract1/2
  Max_Speed/1 -> Subtract1/1
  MaxOutputSpeedSensor/1 -> Subtract/1

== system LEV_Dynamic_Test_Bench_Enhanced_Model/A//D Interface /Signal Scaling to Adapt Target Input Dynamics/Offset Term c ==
  Scaling Coefficent m : Inport
  Anglog_Input_Min : Constant  Value=Anglog_Input_Min
  MinOutputSpeedSensor : Constant  Value=MinOutputSpeedSensor
  Product : Product
  Subtract2 : Sum  Inputs=+-
  "Offset Term c " : Outport
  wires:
  MinOutputSpeedSensor/1 -> Product/1
  Scaling Coefficent m/1 -> Product/2
  Product/1 -> Subtract2/2
  Subtract2/1 -> "Offset Term c "/1
  Anglog_Input_Min/1 -> Subtract2/1

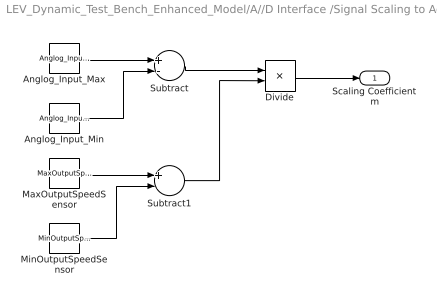
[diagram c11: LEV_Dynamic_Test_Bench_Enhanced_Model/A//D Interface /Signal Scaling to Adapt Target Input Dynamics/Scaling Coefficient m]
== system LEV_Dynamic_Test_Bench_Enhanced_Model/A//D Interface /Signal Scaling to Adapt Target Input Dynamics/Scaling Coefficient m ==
  Anglog_Input_Max : Constant  Value=Anglog_Input_Max
  Anglog_Input_Min : Constant  Value=Anglog_Input_Min
  Divide : Product  Inputs=*/
  MaxOutputSpeedSensor : Constant  Value=MaxOutputSpeedSensor
  MinOutputSpeedSensor : Constant  Value=MinOutputSpeedSensor
  Subtract : Sum  Inputs=+-
  Subtract1 : Sum  Inputs=+-
  Scaling Coefficient m : Outport
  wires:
  Divide/1 -> Scaling Coefficient m/1
  Subtract1/1 -> Divide/2
  Subtract/1 -> Divide/1
  Anglog_Input_Min/1 -> Subtract/2
  MinOutputSpeedSensor/1 -> Subtract1/2
  MaxOutputSpeedSensor/1 -> Subtract1/1
  Anglog_Input_Max/1 -> Subtract/1

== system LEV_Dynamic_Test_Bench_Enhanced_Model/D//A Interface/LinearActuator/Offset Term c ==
  Scaling Coefficent m : Inport
  MinInputBTrq : Constant  Value=MinInputBTrq
  Min_BTrq : Constant  Value=Min_BTrq
  Product : Product
  Subtract2 : Sum  Inputs=+-
  "Offset Term c " : Outport
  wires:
  MinInputBTrq/1 -> Product/1
  Scaling Coefficent m/1 -> Product/2
  Product/1 -> Subtract2/2
  Subtract2/1 -> "Offset Term c "/1
  Min_BTrq/1 -> Subtract2/1

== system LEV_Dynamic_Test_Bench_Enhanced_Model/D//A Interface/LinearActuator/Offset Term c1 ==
  Scaling Coefficent m : Inport
  MinInputBTrq : Constant  Value=MinInputBTrq
  Min_BTrq : Constant  Value=Min_BTrq
  Product : Product
  Subtract2 : Sum  Inputs=+-
  "Offset Term c " : Outport
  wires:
  MinInputBTrq/1 -> Product/1
  Scaling Coefficent m/1 -> Product/2
  Product/1 -> Subtract2/2
  Subtract2/1 -> "Offset Term c "/1
  Min_BTrq/1 -> Subtract2/1

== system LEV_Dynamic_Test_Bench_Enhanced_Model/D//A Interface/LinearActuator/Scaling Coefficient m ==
  Divide : Product  Inputs=*/
  MaxInputBTrq : Constant  Value=MaxInputBTrq
  Max_BTrq : Constant  Value=Max_BTrq
  MinInputBTrq : Constant  Value=MinInputBTrq
  Min_BTrq : Constant  Value=Min_BTrq
  Subtract : Sum  Inputs=+-
  Subtract1 : Sum  Inputs=+-
  Scaling Coefficient m : Outport
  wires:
  Divide/1 -> Scaling Coefficient m/1
  Subtract1/1 -> Divide/2
  Subtract/1 -> Divide/1
  Min_BTrq/1 -> Subtract/2
  MinInputBTrq/1 -> Subtract1/2
  MaxInputBTrq/1 -> Subtract1/1
  Max_BTrq/1 -> Subtract/1

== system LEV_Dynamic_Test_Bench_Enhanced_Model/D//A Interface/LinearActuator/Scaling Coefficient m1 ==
  Divide : Product  Inputs=*/
  MaxInputBTrq : Constant  Value=MaxInputBTrq
  Max_BTrq : Constant  Value=Max_BTrq
  MinInputBTrq : Constant  Value=MinInputBTrq
  Min_BTrq : Constant  Value=Min_BTrq
  Subtract : Sum  Inputs=+-
  Subtract1 : Sum  Inputs=+-
  Scaling Coefficient m : Outport
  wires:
  Divide/1 -> Scaling Coefficient m/1
  Subtract1/1 -> Divide/2
  Subtract/1 -> Divide/1
  Min_BTrq/1 -> Subtract/2
  MinInputBTrq/1 -> Subtract1/2
  MaxInputBTrq/1 -> Subtract1/1
  Max_BTrq/1 -> Subtract/1

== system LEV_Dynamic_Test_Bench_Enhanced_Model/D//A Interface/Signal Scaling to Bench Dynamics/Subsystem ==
  note: Max_Signal-grad1*Digital_Output-offSet1 Min_Signal-Anglog_Input_Min*grad1-offSet1
  Anglog_Output_Max : Constant  Value=Anglog_Output_Max
  Anglog_Output_Min : Constant  Value=Anglog_Output_Min
  Divide : Product  Inputs=/*
  MaxInputBTrq : Constant  Value=MaxInputBTrq
  MinInputBTrq : Constant  Value=MinInputBTrq
  Subtract : Sum  Inputs=+-
  Subtract1 : Sum  Inputs=+-
  "Gradient " : Outport
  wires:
  Divide/1 -> "Gradient "/1
  Subtract1/1 -> Divide/2
  Subtract/1 -> Divide/1
  Anglog_Output_Min/1 -> Subtract/2
  MinInputBTrq/1 -> Subtract1/2
  MaxInputBTrq/1 -> Subtract1/1
  Anglog_Output_Max/1 -> Subtract/1

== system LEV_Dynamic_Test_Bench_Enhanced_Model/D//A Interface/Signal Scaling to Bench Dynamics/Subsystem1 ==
  "Gradient " : Inport
  Anglog_Output_Min : Constant  Value=Anglog_Output_Min
  "MinInputBTrq " : Constant  Value=MinInputBTrq
  Product : Product
  Subtract2 : Sum  Inputs=+-
  "Offset " : Outport
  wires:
  Anglog_Output_Min/1 -> Product/1
  "Gradient "/1 -> Product/2
  Product/1 -> Subtract2/2
  Subtract2/1 -> "Offset "/1
  "MinInputBTrq "/1 -> Subtract2/1

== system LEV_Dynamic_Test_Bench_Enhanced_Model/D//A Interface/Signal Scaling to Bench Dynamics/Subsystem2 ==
  note: Max_Signal-grad1*Digital_Output-offSet1 Min_Signal-Anglog_Input_Min*grad1-offSet1
  Anglog_Output_Max : Constant  Value=Anglog_Output_Max
  Anglog_Output_Min : Constant  Value=Anglog_Output_Min
  Divide : Product  Inputs=/*
  MaxInputBTrq : Constant  Value=MaxInputBTrq
  MinInputBTrq : Constant  Value=MinInputBTrq
  Subtract : Sum  Inputs=+-
  Subtract1 : Sum  Inputs=+-
  "Gradient " : Outport
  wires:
  Divide/1 -> "Gradient "/1
  Subtract1/1 -> Divide/2
  Subtract/1 -> Divide/1
  Anglog_Output_Min/1 -> Subtract/2
  MinInputBTrq/1 -> Subtract1/2
  MaxInputBTrq/1 -> Subtract1/1
  Anglog_Output_Max/1 -> Subtract/1

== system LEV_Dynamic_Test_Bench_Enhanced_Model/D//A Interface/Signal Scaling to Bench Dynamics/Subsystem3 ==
  "Gradient " : Inport
  Anglog_Output_Min : Constant  Value=Anglog_Output_Min
  "MinInputBTrq " : Constant  Value=MinInputBTrq
  Product : Product
  Subtract2 : Sum  Inputs=+-
  "Offset " : Outport
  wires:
  Anglog_Output_Min/1 -> Product/1
  "Gradient "/1 -> Product/2
  Product/1 -> Subtract2/2
  Subtract2/1 -> "Offset "/1
  "MinInputBTrq "/1 -> Subtract2/1
